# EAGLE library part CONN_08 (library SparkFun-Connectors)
Multi connection point. Often used as Generic Header-pin footprint for 0.1 inch spaced/style header connections On any of the 0.1 inch spaced packages, you can populate with these: Break Away Headers - Straight (PRT-00116) Break Away Male Headers - Right Angle (PRT-00553) Female Headers (PRT-00115) Break Away Headers - Machine Pin (PRT-00117) Break Away Female Headers - Swiss Machine Pin (PRT-00743) Arduino Stackable Header - 8 Pin (PRT-09279) For SCREWTERMINALS and SPRING TERMINALS visit here: Screw Terimnals on SparkFun.com (5mm/3.5mm/2.54mm spacing) This device is also useful as a general connection point to wire up your design to another part of your project. Our various solder wires solder well into these plated through hole pads. Hook-Up Wire - Assortment (Stranded, 22 AWG) (PRT-11375) Hook-Up Wire - Assortment (Solid Core, 22 AWG) (PRT-11367) View the entire wire category on our website here Special notes: Molex polarized connector foot print use with SKU : PRT-08231 with associated crimp pins and housings. 1MM SMD Version SKU: PRT-10208 NOTES ON THE VARIANTS LOCK and LOCK_LONGPADS... This footprint was designed to help hold the alignment of a through-hole component (i.e. 6-pin header) while soldering it into place. You may notice that each hole has been shifted either up or down by 0.005 of an inch from it's more standard position (which is a perfectly straight line). This slight alteration caused the pins (the squares in the middle) to touch the edges of the holes.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
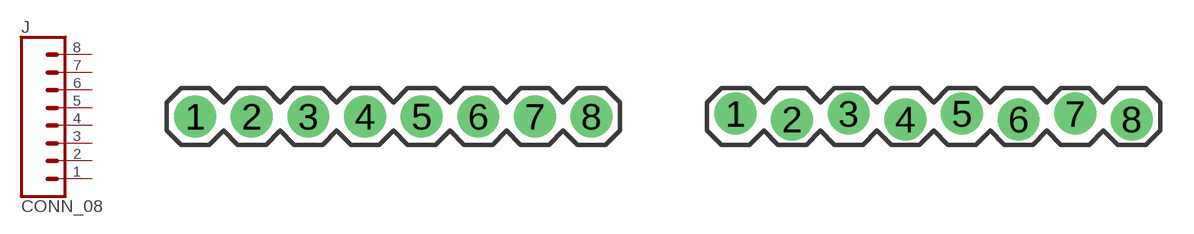
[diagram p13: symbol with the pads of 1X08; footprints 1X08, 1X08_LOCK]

Designator prefix J

## CONN_08" (PROD_ID: CONN-08438)  [1X08]
1  1  pas
2  2  pas
3  3  pas
4  4  pas
5  5  pas
6  6  pas
7  7  pas
8  8  pas

## CONN_08LOCK  [1X08_LOCK]
Pads as for 1X08

## CONN_08LOCK_LONGPADS  [1X08_LOCK_LONGPADS]
Pads as for 1X08

## CONN_08LONGPADS  [1X08_LONGPADS]
Pads as for 1X08

## CONN_083.5MM-8  [SCREWTERMINAL-3.5MM-8]
Pads as for 1X08

## CONN_08SMD-STRAIGHT-FEMALE (PROD_ID: CONN-10204; SF_ID: PRT-11543)  [1X08_SMD]
Pads as for 1X08

## CONN_08SMD-STRAIGHT-ALT-FEMALE (PROD_ID: CONN-10204; SF_ID: PRT-11543)  [1X08_SMD_ALT]
Pads as for 1X08

## CONN_08SMD-COMBO-FEMALE (PROD_ID: CONN-10204; SF_ID: PRT-11543)  [1X08_SMD_COMBINED]
Pads as for 1X08

## CONN_08BM08B-SRSS-TB (PROD_ID: CONN-10556)  [BM08B-SRSS-TB]
Pads as for 1X08

## CONN_08SMD-MALE (PROD_ID: CONN-11292; SF_ID: PRT-11541)  [1X08_SMD_MALE]
Pads as for 1X08

## CONN_08NO_SILK_FEMALE_PTH (PROD_ID: CONN-08438)  [1X08_NO_SILK]
Pads as for 1X08

## CONN_08LOCK_NO_SILK  [1X08_LOCK_NO_SILK]
Pads as for 1X08

## CONN_08FEMALE_LOCK (PROD_ID: CONN-09233; SF_ID: PRT-09279)  [1X08_FEMALE_LOCK]
Pads as for 1X08

## Footprint 1X08 (pad centres in mm)
Plated Through Hole -8 Pin Specifications: Pin count:8 Pin pitch:0.1" Example device(s): CONN_08
drill 1.016 pad 1.88: 1 0,0; 2 2.54,0; 3 5.08,0; 4 7.62,0; 5 10.16,0; 6 12.7,0; 7 15.24,0; 8 17.78,0

## Footprint 1X08_LOCK (pad centres in mm)
Plated Through Hole -8 Pin Locking Footprint Holes are offset 0.005", to hold pins in place during soldering. Specifications: Pin count:8 Pin pitch:0.1" Example device(s): CONN_08
drill 1.016 pad 1.88: 1 0,0.127; 2 2.54,-0.127; 3 5.08,0.127; 4 7.62,-0.127; 5 10.16,0.127; 6 12.7,-0.127; 7 15.24,0.127; 8 17.78,-0.127

## Footprint 1X08_LOCK_LONGPADS (pad centres in mm)
Plated Through Hole -8 Pin Locking Footprint with Long Pads Holes are offset 0.005", to hold pins in place during soldering. Specifications: Pin count:8 Pin pitch:0.1" Example device(s): CONN_08
drill 1.016 long: 1 0,0.127; 2 2.54,-0.127; 3 5.08,0.127; 4 7.62,-0.127; 5 10.16,0.127; 6 12.7,-0.127; 7 15.24,0.127; 8 17.78,-0.127

## Footprint 1X08_LONGPADS (pad centres in mm)
Plated Through Hole -8 Pin Long Pads Specifications: Pin count:8 Pin pitch:0.1" Example device(s): CONN_08
drill 1.118 pad 1.88 long: 1 0,0; 2 2.54,0; 3 5.08,0; 4 7.62,0; 5 10.16,0; 6 12.7,0; 7 15.24,0; 8 17.78,0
